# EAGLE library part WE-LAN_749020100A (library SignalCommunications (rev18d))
WE-LAN LAN Transformer Characteristics Compliant with standards: IEEE 802.3u, IEEE 802.3ab, IEEE 802.3af, IEEE 802.3at and upcoming IEE 802.3bt SMD Applications Ethernet speed up to 10 Gbit/s Power over Ethernet PoE and PoE+ Compliant with most IC’s for Ethernet applications such as Intel, AMD, Microchip and Realtek Hub, Router, Switches, IPcameras, IoT Details see: http://katalog.we-online.de/en/pbs/WE-LAN Created by Yingchun Shan 2016 (C) Wurth Elektronik
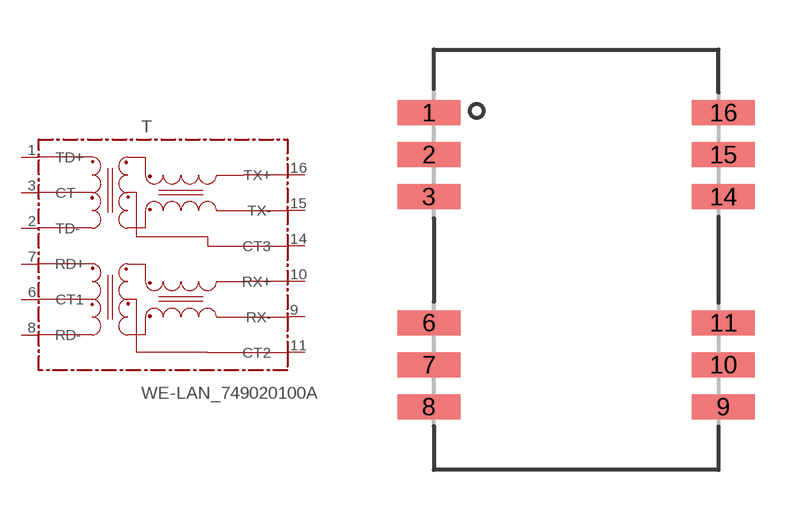
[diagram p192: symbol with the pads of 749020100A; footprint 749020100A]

Designator prefix T

## WE-LAN_749020100A  [749020100A]
1  TD+
2  TD-
3  CT
6  CT1
7  RD+
8  RD-
9  RX-
10  RX+
11  CT2
14  CT3
15  TX-
16  TX+

## Footprint 749020100A (pad centres in mm)
smd 1.9 x 0.76: 1 -4.45,4.445; 2 -4.45,3.175; 3 -4.45,1.905; 6 -4.45,-1.905; 7 -4.45,-3.175; 8 -4.45,-4.445; 9 4.45,-4.445; 10 4.45,-3.175; 11 4.45,-1.905; 14 4.45,1.905; 15 4.45,3.175; 16 4.45,4.445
